TYPE STR_HEATER_LINE_CUS_OUT :
STRUCT
	SBrkAlarm_EN	:	USINT	;
	Temp_Hi_Alarm_Inhibit	:	USINT	;
	Inhibit_Buffer	:	REAL	;
	RateUp	:	REAL	;
	RateDown	:	REAL	;
	PID_P	:	REAL	;
	PID_I	:	REAL	;
	PID_D	:	REAL	;
	AutotuneActivate	:	USINT	;
	Autotune_PID_Sel:USINT;
END_STRUCT
END_TYPE
